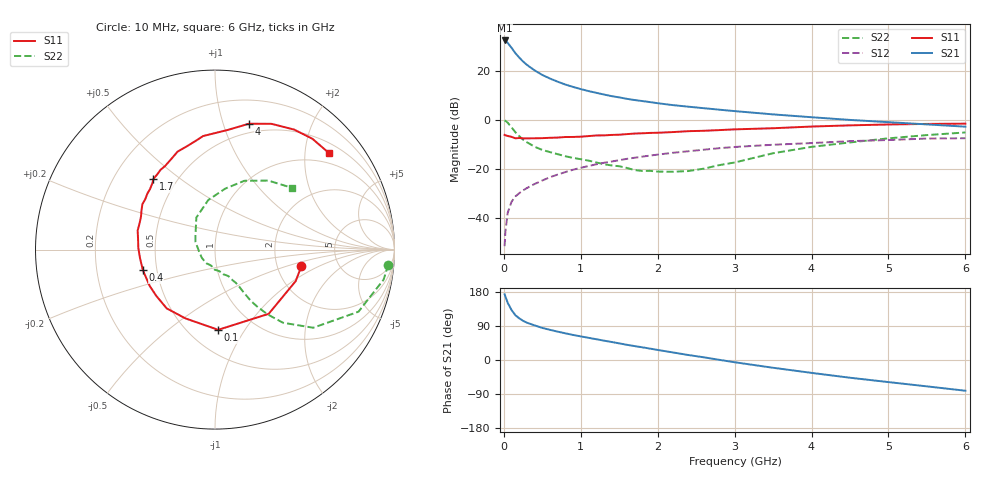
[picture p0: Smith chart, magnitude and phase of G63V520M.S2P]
! SIEMENS Small Signal Semiconductors
! BFG193
! Si NPN RF Bipolar Junction Transistor in SOT223
! VCE = 3.5 V  IC = 20 mA
! Common Emitter S-Parameters:  August  1996
# GHz  S  MA  R  50
!  f  S11  S21  S12  S22
! GHz  MAG  ANG  MAG  ANG  MAG  ANG  MAG  ANG
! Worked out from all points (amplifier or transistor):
!   36 points, 10 MHz to 6 GHz, reference 50 ohm
!   highest |S21| = 32.4 dB at 10 MHz (marker M1)
!   |S21| within 3 dB of that: start of sweep to 99.61 MHz
!   unconditionally stable (mu >= 1): 672 MHz to 2.411 GHz
!   at 250 MHz: K = 0.74, MSG = 26.4 dB, |S12| = -28.9 dB
!   at 1.4 GHz: K = 1.05, MAG = 12.0 dB, |S12| = -17.1 dB
!   at 6 GHz: K = 0.89, MSG = 2.4 dB, |S12| = -7.5 dB
!   S11 on the Smith chart (normalised r, x): 10 MHz: 2.73, -0.67; 100 MHz: 0.69, -0.77; 400 MHz: 0.42, -0.12; 1.7 GHz: 0.37, +0.40; 4 GHz: 0.41, +1.22; 6 GHz: 0.73, +2.56
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0.01  0.4901 -11.0  41.85 173.4  0.0026 87.9  0.9692 -5.0
0.02  0.4825 -21.4  41.25 168.0  0.0051 82.4  0.9541 -10.1
0.05  0.4664 -50.1  37.4 150.8  0.0125 70.5  0.8712 -23.4
0.1  0.4473 -87.7  29.57 132.0  0.0211 63.8  0.6993 -38.5
0.15  0.4172 -113.2  23.05 118.1  0.027 59.0  0.5561 -47.1
0.2  0.424 -129.4  18.73 110.0  0.0315 58.8  0.4634 -51.0
0.25  0.4165 -142.0  15.54 103.4  0.0359 58.5  0.3918 -53.6
0.3  0.4164 -150.9  13.26 98.5  0.0402 59.3  0.3471 -55.1
0.4  0.418 -164.1  10.23 91.3  0.0486 60.1  0.2807 -56.3
0.5  0.4209 -174.1  8.246 84.7  0.0573 60.0  0.2416 -56.9
0.6  0.4274 178.6  6.961 79.6  0.067 60.2  0.218 -57.9
0.7  0.4324 172.4  6.002 74.8  0.0757 59.7  0.1978 -60.0
0.9  0.4449 161.1  4.691 66.1  0.0951 57.9  0.166 -63.0
1.1  0.4635 152.1  3.862 58.6  0.113 55.4  0.1461 -71.0
1.4  0.4894 140.3  3.044 47.6  0.1399 50.1  0.1165 -84.1
1.7  0.5223 131.0  2.532 36.7  0.1672 44.5  0.0934 -101.6
2.2  0.5602 115.8  1.99 19.9  0.2113 33.9  0.0865 -148.4
3.5  0.671 83.8  1.288 -20.5  0.3083 3.7  0.2066 120.2
4  0.7265 74.9  1.127 -34.0  0.3337 -5.9  0.2789 97.7
4.5  0.7682 65.8  0.992 -46.8  0.3651 -16.2  0.3439 80.6
5.5  0.8221 48.7  0.804 -69.6  0.4127 -39.6  0.486 52.3
6  0.8325 40.1  0.722 -81.1  0.4195 -53.0  0.55 38.7
